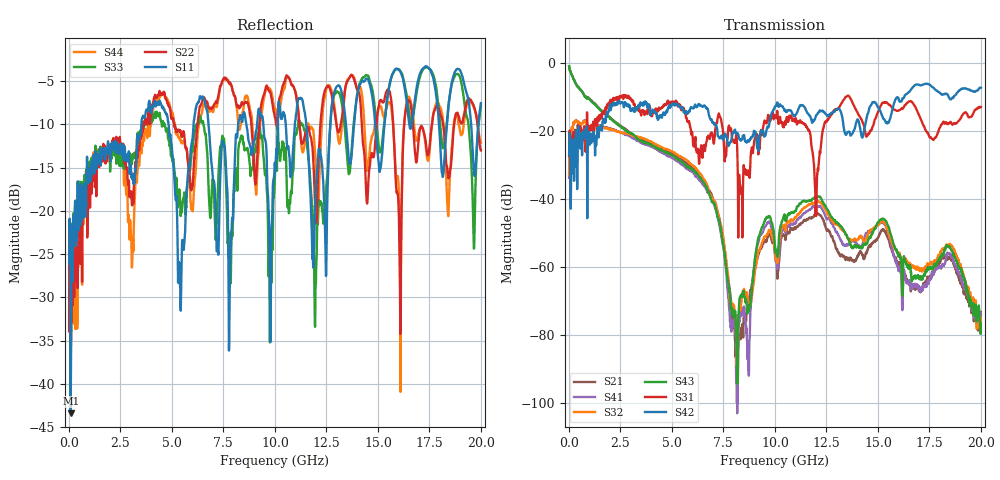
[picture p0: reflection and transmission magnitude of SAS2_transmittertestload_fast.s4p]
! SAS 2.0 test load s-parameter file, representing performance of the
! Molex miniSAS 10-meter cable assembly.
! Model includes test fixture effects, comprised of trace loss (55 mm of
! 7-mil single-ended stripline trace in 4000-13 PC board material) and
! connector SMT attach.
!	Modified from SAS2_transmittertestload by multiplying S12, S14,
!	S21, S23, S32, S34, S41 & S43 by exp(j*2pi*freq*delay), where
!	delay is about 45 ns, in order to minimize cable delay.  This
!	minimizes number of required frequency steps.
!  Mike Jenkins	11May07
! Frequency range of coverage is 10 MHz to 20 GHz, in 10 MHz steps.
! Model Node Map:
! Input port (pin)	Output port (pin)
! 1 (B5)		2 (A5)
! 3 (B6)		4 (A6)
# MHz S MA R 50.00
! FREQ  S11  S12  S13  S14
!  S21  S22  S23  S24
!  S31  S32  S33  S34
!  S41  S42  S43  S44
!  MAG  ANG  MAG  ANG  MAG  ANG  MAG  ANG
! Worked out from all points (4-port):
!   2000 points, 10 MHz to 20 GHz, reference 50 ohm
!   strongest paths, dB at 10 MHz, 5.01 GHz, 10.01 GHz, 15.01 GHz, 20 GHz:
!     S42: -27.1, -12.0, -12.8, -13.2, -7.4
!     S31: -27.4, -11.4, -16.2, -14.4, -13.1
!     S43: -1.0, -27.3, -54.5, -46.9, -76.6
!     S32: -33.1, -26.1, -56.3, -47.8, -75.2
!     S41: -33.8, -28.1, -57.1, -47.4, -76.1
!     S21: -1.1, -26.6, -56.3, -51.5, -73.9
!   lowest |S11| = -43.4 dB at 90 MHz (marker M1), VSWR 1.01, Z = 50.2 + j0.657 ohm
!   |S11| at or under -10 dB: start of sweep to 3.519 GHz; 4.839 GHz to 6.051 GHz (1.212 GHz wide, 22.3 % of centre); 6.783 GHz to 8.217 GHz (1.433 GHz wide, 19.1 % of centre)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
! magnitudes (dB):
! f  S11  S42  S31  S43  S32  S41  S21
! 10 MHz  -26.1  -27.1  -27.4  -1.0  -33.1  -33.8  -1.1
! 90 MHz  -43.4  -42.9  -41.6  -2.8  -22.3  -22.3  -2.7
! 6.18 GHz  -8.0  -13.0  -25.4  -32.4  -31.2  -33.5  -32.4
! 8.15 GHz  -11.5  -20.8  -22.4  -86.6  -86.4  -94.4  -93.2
! 12.1 GHz  -13.8  -14.8  -31.6  -39.3  -40.8  -42.2  -44.4
! 13.5 GHz  -11.3  -20.7  -9.8  -51.1  -51.3  -53.4  -57.6
! 20 GHz  -7.5  -7.4  -13.1  -76.6  -75.2  -76.1  -73.9
